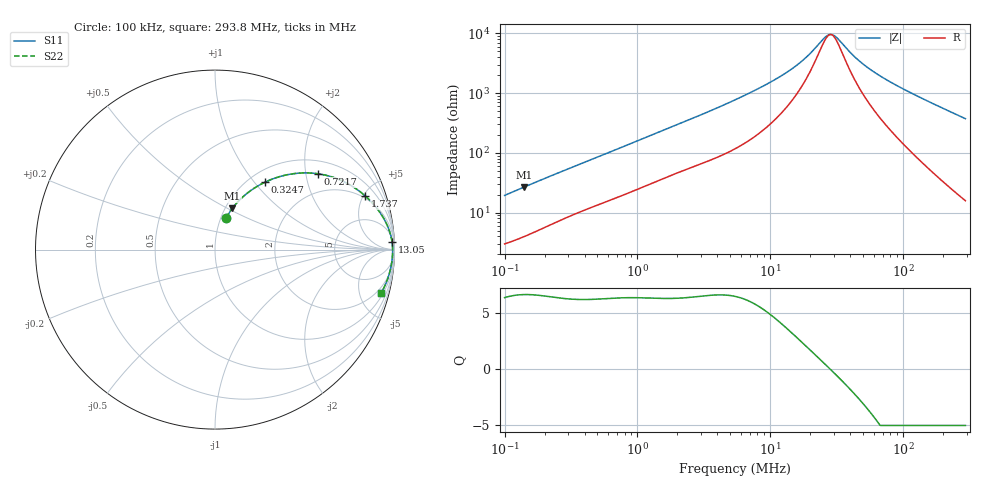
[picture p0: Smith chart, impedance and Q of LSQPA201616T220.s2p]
! LSQPA201616T220  S-PARAMETER MODEL  ( General Type )
! Model Generated by TAIYO YUDEN Corporation (http://www.ty-top.com)
! Version 2.0
! TAIYO YUDEN Control No. 100810NF25SB-FKC
! Copyright(c) 2007 TAIYO YUDEN CO.,LTD. All Rights Reserved.
! Product Description (link to TY-COMPAS)
! https://ds.yuden.co.jp/TYCOMPAS/or/detail?pn=LSQPA201616T220K&u=M
! Products Name : Inductors
! Characteristics :
!  Inductance : 22 uH , SRF(min) : 16 MHz , DC Resistance(max) : 2.34 Ohm
!  Rated Current : Saturation :250 mA , Temp Rise : 240 mA (40 degC)
!  Case Size : 2.0 x 1.6 / 0.079 x 0.063 [mm/inch] , Thickness : 1.6 / 0.063 [mm/inch]
!  (Conditions: Temperature = 25 degC , DC Bias Current/Voltage = 0A / 0V)
! External Node Assignments :
!  1  o---GGG---o  2
! GND o---------o GND
! Frequency Range : 0.1MHz  -  293.796821MHz  [ 402 STEP ]
# MHz S RI R 50
! Freq[MHz].  S11 Real  S11 Imag  S21 Real  S21 Imag  S12 Real  S12 Imag  S22 Real  S22 Imag
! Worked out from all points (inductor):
!   401 points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, 100 kHz to 293.8 MHz, reference 50 ohm
!   read as one part in series: L = 30.1 uH near 104.1 kHz
!   highest Q = 6.69 at 140.4 kHz (marker M1), where L = 30 uH
!   self-resonance near 28.38 MHz
!   S11 on the Smith chart (normalised r, x): 100 kHz: 1.06, +0.38; 324.7 kHz: 1.18, +1.14; 721.7 kHz: 1.37, +2.34; 1.737 MHz: 1.82, +5.18; 13.05 MHz: 12, +42; 293.8 MHz: 1.32, -7.48
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0.1  0.0614 0.1744  0.9386 -0.1744  0.9386 -0.1744  0.0614 0.1744
0.140408  0.0967 0.2301  0.9033 -0.2301  0.9033 -0.2301  0.0967 0.2301
0.213533  0.1696 0.3063  0.8304 -0.3063  0.8304 -0.3063  0.1696 0.3063
0.324741  0.2802 0.3764  0.7198 -0.3764  0.7198 -0.3764  0.2802 0.3764
0.380976  0.332 0.3976  0.668 -0.3976  0.668 -0.3976  0.332 0.3976
0.721675  0.5723 0.4226  0.4277 -0.4226  0.4277 -0.4226  0.5723 0.4226
1.451429  0.798 0.3304  0.202 -0.3304  0.202 -0.3304  0.798 0.3304
1.737108  0.838 0.2979  0.162 -0.2979  0.162 -0.2979  0.838 0.2979
2.919106  0.9183 0.2078  0.0817 -0.2078  0.0817 -0.2078  0.9183 0.2078
5.420303  0.9655 0.1213  0.0345 -0.1213  0.0345 -0.1213  0.9655 0.1213
8.928459  0.9812 0.0714  0.0188 -0.0714  0.0188 -0.0714  0.9812 0.0714
13.04694  0.9864 0.0433  0.0136 -0.0433  0.0136 -0.0433  0.9864 0.0433
16.91298  0.9883 0.0275  0.0117 -0.0275  0.0117 -0.0275  0.9883 0.0275
20.65007  0.9891 0.0165  0.0109 -0.0165  0.0109 -0.0165  0.9891 0.0165
26.23994  0.9896 0.00401  0.0104 -0.00401  0.0104 -0.00401  0.9896 0.00401
29.579  0.9897 -0.0021  0.0103 0.0021  0.0103 0.0021  0.9897 -0.0021
32.0379  0.9898 -0.00618  0.0102 0.00618  0.0102 0.00618  0.9898 -0.00618
40.71041  0.9896 -0.0188  0.0104 0.0188  0.0104 0.0188  0.9896 -0.0188
48.72328  0.9891 -0.0289  0.0109 0.0289  0.0109 0.0289  0.9891 -0.0289
78.67184  0.9862 -0.0613  0.0138 0.0613  0.0138 0.0613  0.9862 -0.0613
143.1934  0.9746 -0.1217  0.0254 0.1217  0.0254 0.1217  0.9746 -0.1217
293.7968  0.9245 -0.244  0.0755 0.244  0.0755 0.244  0.9245 -0.244
